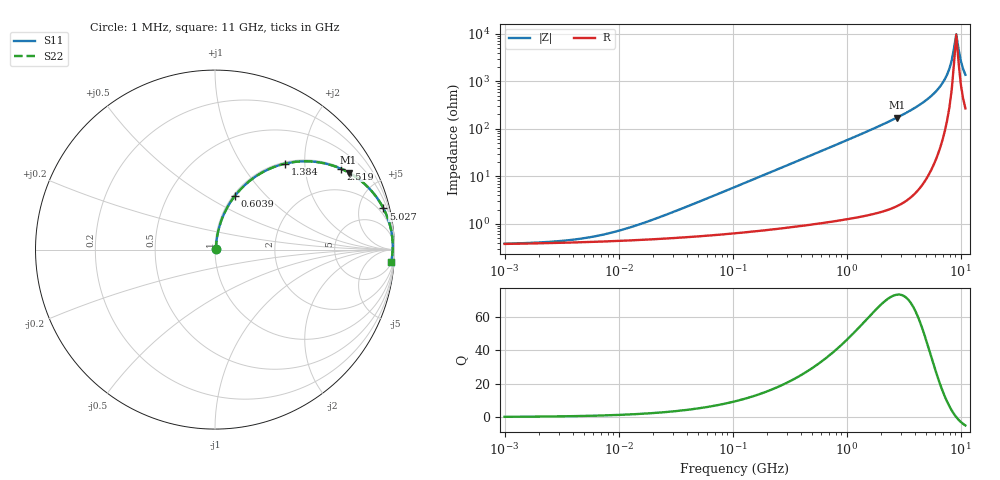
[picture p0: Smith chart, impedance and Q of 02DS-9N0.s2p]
# MHz S MA R 50
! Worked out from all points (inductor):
!   203 points, 1 MHz to 11 GHz, reference 50 ohm
!   read as one part in series: L = 9 nH near 26.33 MHz
!   highest Q = 72.9 at 2.762 GHz (marker M1), where L = 9.9 nH
!   self-resonance near 8.737 GHz
!   S11 on the Smith chart (normalised r, x): 1 MHz: 1.01, +0.00; 603.9 MHz: 1.02, +0.69; 1.384 GHz: 1.03, +1.60; 2.519 GHz: 1.04, +3.08; 5.027 GHz: 1.18, +8.15; 11 GHz: 6, -27
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1  0.003803 8.5  0.9962 -0.0  0.9962 -0.0  0.003803 8.5
4.78889  0.004895 33.3  0.9959 -0.2  0.9959 -0.2  0.004895 33.3
10.0079  0.007119 52.0  0.9956 -0.3  0.9956 -0.3  0.007119 52.0
22.9334  0.01377 68.9  0.9951 -0.7  0.9951 -0.7  0.01377 68.9
104.881  0.05917 80.5  0.992 -3.4  0.992 -3.4  0.05917 80.5
240.337  0.134 79.0  0.9834 -7.7  0.9834 -7.7  0.134 79.0
502.263  0.2717 72.3  0.9532 -15.8  0.9532 -15.8  0.2717 72.3
603.891  0.3216 69.5  0.9373 -18.8  0.9373 -18.8  0.3216 69.5
914.156  0.4587 61.4  0.8781 -27.3  0.8781 -27.3  0.4587 61.4
1383.83  0.6198 50.7  0.7737 -38.3  0.7737 -38.3  0.6198 50.7
2405.28  0.82 34.1  0.5611 -55.1  0.5611 -55.1  0.82 34.1
2518.67  0.8337 32.7  0.5408 -56.5  0.5408 -56.5  0.8337 32.7
2761.76  0.8593 30.0  0.4999 -59.2  0.4999 -59.2  0.8593 30.0
3812.71  0.9291 20.8  0.356 -68.3  0.356 -68.3  0.9291 20.8
5026.61  0.9662 13.7  0.2372 -75.0  0.2372 -75.0  0.9662 13.7
6328.63  0.9835 8.2  0.1433 -79.3  0.1433 -79.3  0.9835 8.2
7609.17  0.9898 4.1  0.0712 -79.7  0.0712 -79.7  0.9898 4.1
8343.56  0.9905 2.0  0.03635 -73.9  0.03635 -73.9  0.9905 2.0
9148.82  0.9898 -0.0  0.01024 0.0  0.01024 0.0  0.9898 -0.0
9580.14  0.9888 -1.0  0.02076 56.8  0.02076 56.8  0.9888 -1.0
10031.8  0.9874 -2.0  0.0371 69.2  0.0371 69.2  0.9874 -2.0
11000  0.9835 -4.0  0.07161 74.7  0.07161 74.7  0.9835 -4.0
